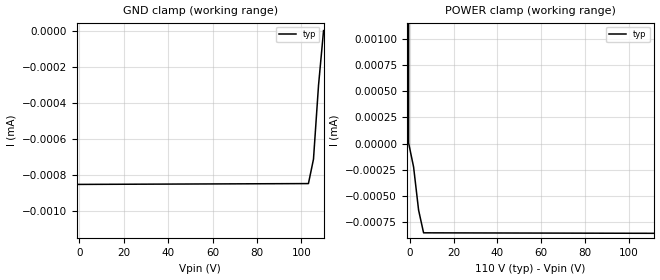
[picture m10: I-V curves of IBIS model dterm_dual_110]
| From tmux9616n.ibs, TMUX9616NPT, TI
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| dterm_dual_110
[Model]   dterm_dual_110
Model_type   Terminator
|   typ   min   max
C_comp   6.362683e-12   NA   NA
[Voltage Range]   110   NA   NA
[Temperature Range]   27   NA   NA
[Power Clamp Reference]   110   NA   NA
[GND Clamp Reference]   0   NA   NA
[GND Clamp]
|   Voltage   I(typ)   I(min)   I(max)
-115V     -1.536A    NA         NA
-112.7V   -584mA     NA         NA
-110.5V   -878.7nA   NA         NA
-108.2V   -858.4nA   NA         NA
103.2V    -849.1nA   NA         NA
105.5V    -713.9nA   NA         NA
107.7V    -303.5nA   NA         NA
110V      1.104nA    NA         NA
[POWER Clamp]
|   Voltage   I(typ)   I(min)   I(max)
-5V       1.098A     NA         NA
-2.727V   449.9mA    NA         NA
-455mV    6.952nA    NA         NA
1.818V    -221.6nA   NA         NA
4.091V    -632.1nA   NA         NA
6.364V    -849.1nA   NA         NA
220V      -858.5nA   NA         NA
